(* Logix 5000 AddOnInstructionDefinition export AMCI_3202_AOP_Preset; software revision 20.03 *)

ADD_ON_INSTRUCTION AMCI_3202_AOP_Preset   (* revision 1.0, vendor AMCI, ExecuteEnableInFalse *)
VAR_INPUT
   axis_status_bits : INT; {required}
   channel_number : INT; {required}
   Target_Position : DINT; {required}
END_VAR
VAR_IN_OUT
   AMCI_3202_output_data : AM:1756_3202:O:0; {required}
END_VAR
VAR_OUTPUT
   EN : BOOL; {access Read Only, visible}
   ER : BOOL; {access Read Only, visible}
END_VAR
VAR
   command_data_block : DINT[8]; {access None}
END_VAR

ROUTINE EnableInFalse   (* ladder *)
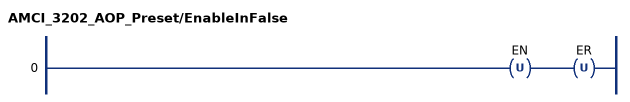
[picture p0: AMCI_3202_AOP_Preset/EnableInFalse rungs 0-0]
   0: OTU(EN)OTU(ER);
END_ROUTINE

ROUTINE Logic   (* ladder *)
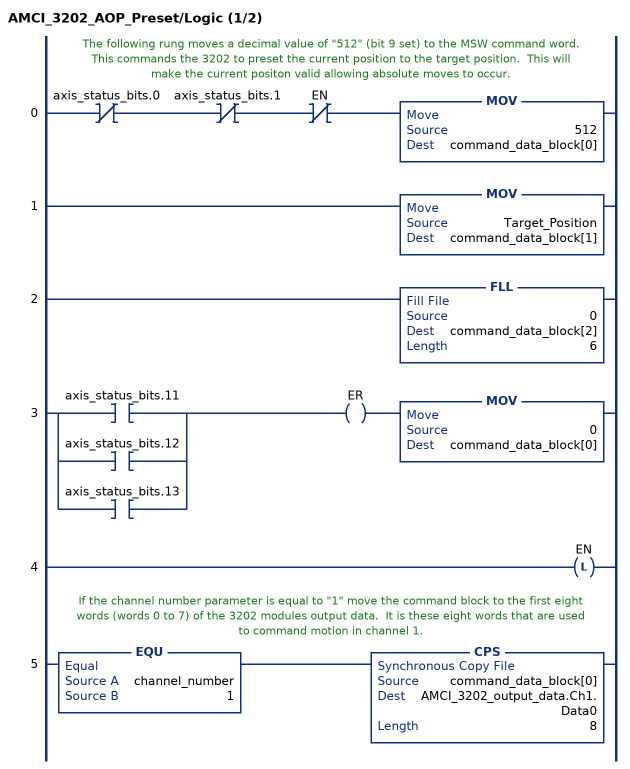
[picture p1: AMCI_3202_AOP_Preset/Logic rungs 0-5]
   // The following rung moves a decimal value of "512" (bit 9 set) to the MSW command word.  This commands the 3202 to preset the current position to the target position.  This will make the current positon valid allowing absolute moves to occur.
   0: XIO(axis_status_bits.0)XIO(axis_status_bits.1)XIO(EN)MOV(512,command_data_block[0]);
   1: MOV(Target_Position,command_data_block[1]);
   2: FLL(0,command_data_block[2],6);
   3: [XIC(axis_status_bits.11) ,XIC(axis_status_bits.12) ,XIC(axis_status_bits.13) ]OTE(ER)MOV(0,command_data_block[0]);
   4: OTL(EN);
   // If the channel number parameter is equal to "1" move the command block to the first eight words (words 0 to 7) of the 3202 modules output data.  It is these eight words that are used to command motion in channel 1.
   5: EQU(channel_number,1)CPS(command_data_block[0],AMCI_3202_output_data.Ch1.Data0,8);
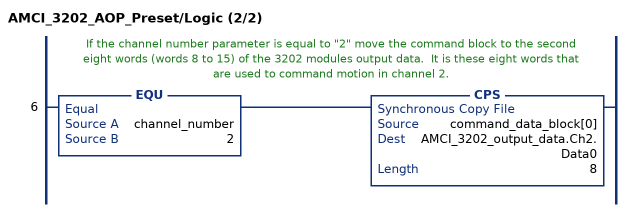
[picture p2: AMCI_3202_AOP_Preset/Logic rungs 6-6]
   // If the channel number parameter is equal to "2" move the command block to the second eight words (words 8 to 15) of the 3202 modules output data.  It is these eight words that are used to command motion in channel 2.
   6: EQU(channel_number,2)CPS(command_data_block[0],AMCI_3202_output_data.Ch2.Data0,8);
END_ROUTINE
END_ADD_ON_INSTRUCTION
